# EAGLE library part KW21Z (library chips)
NXP KW21Z Cortex M0+ 802.15.4
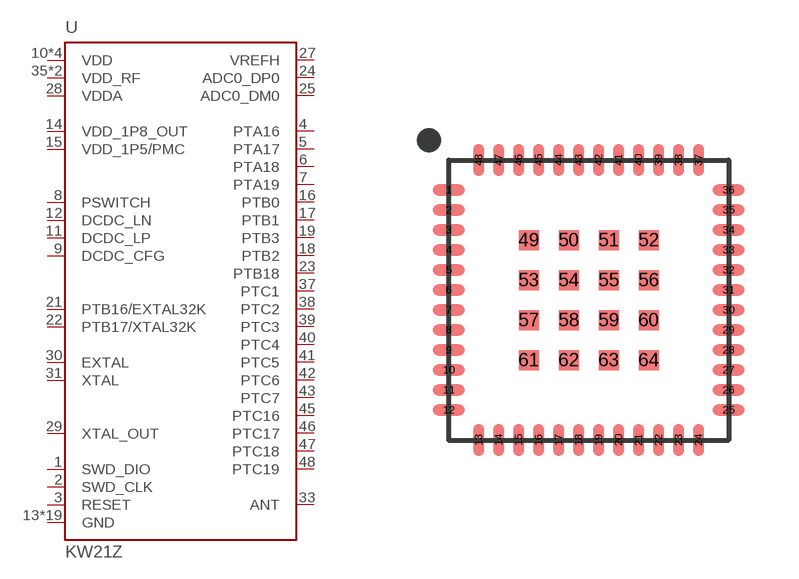
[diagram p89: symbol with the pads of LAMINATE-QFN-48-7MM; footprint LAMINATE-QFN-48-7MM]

Designator prefix U

## KW21Z (DIGIKEY: MKW21Z256VHT4-ND; MPN: MKW21Z256VHT4)  [LAMINATE-QFN-48-7MM]
1  SWD_DIO
2  SWD_CLK
3  RESET
4  PTA16
5  PTA17
6  PTA18
7  PTA19
8  PSWITCH
9  DCDC_CFG
10  VDD
11  DCDC_LP
12  DCDC_LN
13  GND
14  VDD_1P8_OUT
15  VDD_1P5/PMC
16  PTB0
17  PTB1
18  PTB2
19  PTB3
20  VDD
21  PTB16/EXTAL32K
22  PTB17/XTAL32K
23  PTB18
24  ADC0_DP0
25  ADC0_DM0
26  GND
27  VREFH
28  VDDA
29  XTAL_OUT
30  EXTAL
31  XTAL
32  VDD
33  ANT
34  GND
35  VDD_RF
36  VDD_RF
37  PTC1
38  PTC2
39  PTC3
40  PTC4
41  PTC5
42  PTC6
43  PTC7
44  VDD
45  PTC16
46  PTC17
47  PTC18
48  PTC19
49  GND
50  GND
51  GND
52  GND
53  GND
54  GND
55  GND
56  GND
57  GND
58  GND
59  GND
60  GND
61  GND
62  GND
63  GND
64  GND

## Footprint LAMINATE-QFN-48-7MM (pad centres in mm)
7MM x 7MM 48 QFN package
smd 0.8 x 0.28: 1 -3.5,2.75; 2 -3.5,2.25; 3 -3.5,1.75; 4 -3.5,1.25; 5 -3.5,0.75; 6 -3.5,0.25; 7 -3.5,-0.25; 8 -3.5,-0.75; 9 -3.5,-1.25; 10 -3.5,-1.75; 11 -3.5,-2.25; 12 -3.5,-2.75; 25 3.5,-2.75; 26 3.5,-2.25; 27 3.5,-1.75; 28 3.5,-1.25; 29 3.5,-0.75; 30 3.5,-0.25; 31 3.5,0.25; 32 3.5,0.75; 33 3.5,1.25; 34 3.5,1.75; 35 3.5,2.25; 36 3.5,2.75
smd 0.28 x 0.8: 13 -2.75,-3.5; 14 -2.25,-3.5; 15 -1.75,-3.5; 16 -1.25,-3.5; 17 -0.75,-3.5; 18 -0.25,-3.5; 19 0.25,-3.5; 20 0.75,-3.5; 21 1.25,-3.5; 22 1.75,-3.5; 23 2.25,-3.5; 24 2.75,-3.5; 37 2.75,3.5; 38 2.25,3.5; 39 1.75,3.5; 40 1.25,3.5; 41 0.75,3.5; 42 0.25,3.5; 43 -0.25,3.5; 44 -0.75,3.5; 45 -1.25,3.5; 46 -1.75,3.5; 47 -2.25,3.5; 48 -2.75,3.5
smd 0.5 x 0.5: 49 -1.5,1.5; 50 -0.5,1.5; 51 0.5,1.5; 52 1.5,1.5; 53 -1.5,0.5; 54 -0.5,0.5; 55 0.5,0.5; 56 1.5,0.5; 57 -1.5,-0.5; 58 -0.5,-0.5; 59 0.5,-0.5; 60 1.5,-0.5; 61 -1.5,-1.5; 62 -0.5,-1.5; 63 0.5,-1.5; 64 1.5,-1.5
